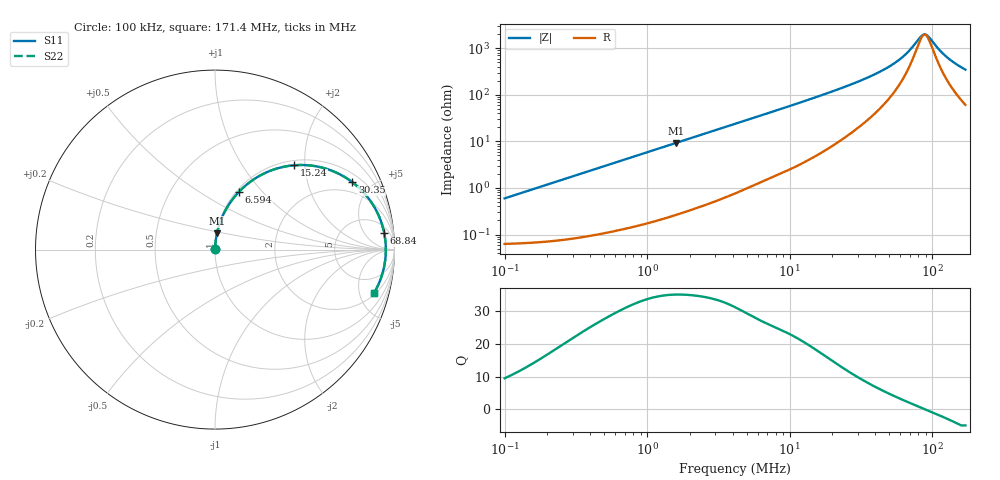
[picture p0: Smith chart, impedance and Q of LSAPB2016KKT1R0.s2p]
! LSAPB2016KKT1R0  S-PARAMETER MODEL  ( General Type )
! Model Generated by TAIYO YUDEN Corporation (http://www.ty-top.com)
! Version 2.0
! TAIYO YUDEN Control No. 20210629
! Copyright(c) 2015 TAIYO YUDEN CO.,LTD. All Rights Reserved.
! Product Description (link to TY-COMPAS)
! https://ds.yuden.co.jp/TYCOMPAS/or/detail?pn=LSAPB2016KKT1R0M&u=M
! Products Name : Inductors
! Characteristics :
!  Inductance : 1.0 uH , SRF(min) : -Hz , DC Resistance(max) : 0.07 Ohm
!  Rated Current : Saturation :2700 mA , Temp Rise : 2300 mA (40 degC)
!  Case Size : 2.0 x 1.6 / 0.079 x 0.063 [mm/inch] , Thickness : 1 / 0.039 [mm/inch]
!  (Conditions: Temperature = 25 degC , DC Bias Current/Voltage = 0A / 0V)
! External Node Assignments :
!  1  o---GGG---o  2
! GND o---------o GND
! Frequency Range : 0.1MHz  -  171.398534MHz  [ 402 STEP ]
# MHz S RI R 50
! Freq[MHz].  S11 Real  S11 Imag  S21 Real  S21 Imag  S12 Real  S12 Imag  S22 Real  S22 Imag
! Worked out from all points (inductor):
!   401 points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, 100 kHz to 171.4 MHz, reference 50 ohm
!   read as one part in series: L = 944 nH near 103.8 kHz
!   highest Q = 35.1 at 1.602 MHz (marker M1), where L = 923 nH
!   self-resonance near 88.73 MHz
!   S11 on the Smith chart (normalised r, x): 100 kHz: 1.00, +0.01; 6.594 MHz: 1.03, +0.75; 15.24 MHz: 1.10, +1.77; 30.35 MHz: 1.39, +3.83; 68.84 MHz: 9, +16; 171.4 MHz: 2.22, -6.85
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0.1  0.000663 0.00593  0.9993 -0.00593  0.9993 -0.00593  0.000663 0.00593
0.348094  0.00129 0.0205  0.9987 -0.0205  0.9987 -0.0205  0.00129 0.0205
1.211692  0.00695 0.0699  0.993 -0.0699  0.993 -0.0699  0.00695 0.0699
1.602019  0.0111 0.0917  0.9889 -0.0917  0.9889 -0.0917  0.0111 0.0917
4.140031  0.0599 0.2218  0.9401 -0.2218  0.9401 -0.2218  0.0599 0.2218
6.593697  0.1337 0.3221  0.8663 -0.3221  0.8663 -0.3221  0.1337 0.3221
9.747974  0.2469 0.4103  0.7531 -0.4103  0.7531 -0.4103  0.2469 0.4103
14.41119  0.4151 0.4671  0.5849 -0.4671  0.5849 -0.4671  0.4151 0.4671
15.23894  0.4425 0.4701  0.5575 -0.4701  0.5575 -0.4701  0.4425 0.4701
21.30517  0.6103 0.4532  0.3897 -0.4532  0.3897 -0.4532  0.6103 0.4532
30.34593  0.7656 0.3753  0.2344 -0.3753  0.2344 -0.3753  0.7656 0.3753
40.12137  0.855 0.286  0.145 -0.286  0.145 -0.286  0.855 0.286
50.16444  0.9039 0.2069  0.0961 -0.2069  0.0961 -0.2069  0.9039 0.2069
59.31453  0.9285 0.1462  0.0715 -0.1462  0.0715 -0.1462  0.9285 0.1462
68.84006  0.9427 0.0921  0.0573 -0.0921  0.0573 -0.0921  0.9427 0.0921
84.48438  0.9516 0.0178  0.0484 -0.0178  0.0484 -0.0178  0.9516 0.0178
91.01574  0.9518 -0.00923  0.0482 0.00923  0.0482 0.00923  0.9518 -0.00923
96.24353  0.9511 -0.0295  0.0489 0.0295  0.0489 0.0295  0.9511 -0.0295
111.6996  0.9446 -0.0836  0.0554 0.0836  0.0554 0.0836  0.9446 -0.0836
124.8998  0.9356 -0.1242  0.0644 0.1242  0.0644 0.1242  0.9356 -0.1242
147.6818  0.9146 -0.1853  0.0854 0.1853  0.0854 0.1853  0.9146 -0.1853
171.3985  0.8877 -0.2391  0.1123 0.2391  0.1123 0.2391  0.8877 -0.2391
